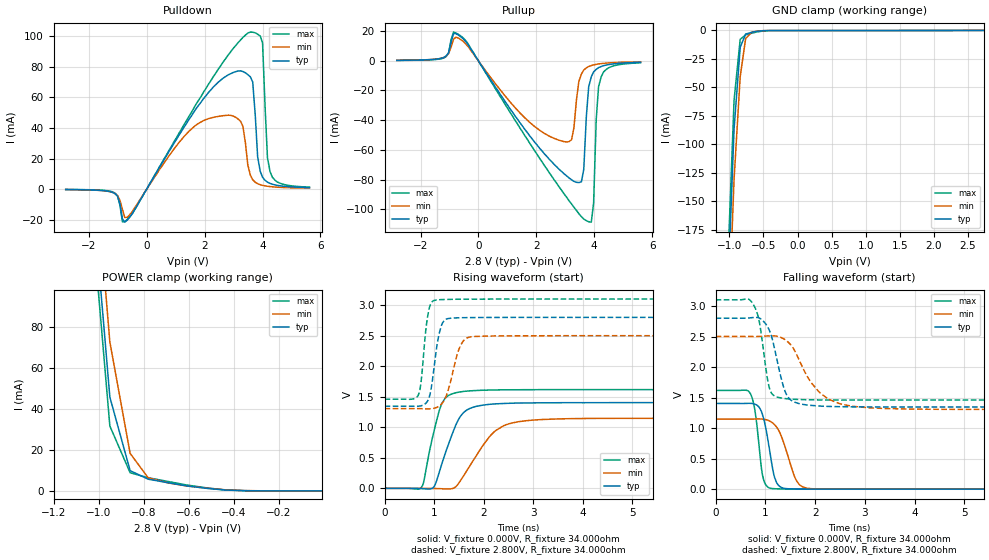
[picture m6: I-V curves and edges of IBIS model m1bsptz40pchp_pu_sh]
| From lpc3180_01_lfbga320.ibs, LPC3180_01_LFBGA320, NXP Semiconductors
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| |   Rev 0.20 IBIS Model Design Automation Generation   |
| |   N O N - S I L I C O N   C O R R E L A T E D   |
| |   This IBIS [Model] is pre-Beta tactical support   |
| |  Note: this IBIS [Model] contains clamp curves generated   |
| |   through simulation which should not be relied upon   |
| mem1bsptz40pchp
|   Bidirectional Pad 2.8
|   3state Output
|   Plain Input
|   1ns Slew Rate control
|   CMOS
| Pull Up Mode (p1=0, p2=0)
[Model]   m1bsptz40pchp_pu_sh | of mem1bsptz40pchp
Model_type   I/O
Polarity   Non-Inverting
Enable   Active-Low
|  Reciever Thresholds
Vinl   = 0.36V
Vinh   = 0.84V
| AC Test Load Conditions
Vref   = 0
Cref   = 1.2e-11
Rref   = 1000000000
Vmeas   = 0.6
| [Process Range]   typical   min   max
| C_comp edge width   400.000ps   400.000ps   400.000ps
| C_comp Tstrobe   40.000fs   40.000fs   40.000fs
C_comp   2.019pF   1.948pF   2.109pF
[Temperature Range]   25   125   -40
[Voltage Range]   2.80V   2.50V   3.10V
[GND Clamp Reference]   0.00V   0.00V   0.00V
[Pulldown Reference]   0.00V   0.00V   0.00V
[POWER Clamp Reference]   2.80V   2.50V   3.10V
[Pullup Reference]   2.80V   2.50V   3.10V
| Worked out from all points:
|   slope of the pulldown table from 0 to 0.42 V, typ, clamps not added: 30.8 ohm
|   slope of the pullup table from 0 to 0.42 V, typ, clamps not added: 32.9 ohm
|   GND clamp passes 1 mA (typ) near -0.61 V on its own axis
|   POWER clamp passes 1 mA (typ) near -0.49 V on its own axis
|   rising waveform, V_fixture 0.000V, R_fixture 34.000ohm: 20-80 % time 380ps typ, 589ps min, 272ps max; typ from 0.001 V to 1.4 V
|   falling waveform, V_fixture 0.000V, R_fixture 34.000ohm: 20-80 % time 183ps typ, 282ps min, 135ps max; typ from 1.4 V to 0.001 V
|   rising waveform, V_fixture 2.800V, R_fixture 34.000ohm: 20-80 % time 155ps typ, 236ps min, 118ps max; typ from 1.35 V to 2.8 V
|   falling waveform, V_fixture 2.800V, R_fixture 34.000ohm: 20-80 % time 260ps typ, 556ps min, 175ps max; typ from 2.8 V to 1.35 V
[GND Clamp]
| ref voltage   0.00V   0.00V   0.00V
|   Voltage   I(typ)   I(min)   I(max)
-2.8V     -3.643A    -3.653A    -3.644A
-1.01V    -211.8mA   -255.9mA   -186.6mA
-930mV    -86.61mA   -130.6mA   -61.25mA
-840mV    -14.85mA   -40.65mA   -7.873mA
-760mV    -3.232mA   -7.1mA     -3.891mA
-670mV    -1.663mA   -1.71mA    -2.461mA
-500mV    -316uA     -247.5uA   -559.8uA
2.73V     -11.67uA   31.94uA    -74.22uA
[Power Clamp]   | Vtable = Vcc - Vpad
| ref voltage   2.80V   2.50V   3.10V
|   Voltage   I(typ)   I(min)   I(max)
-2.82V    3.531A     3.518A     3.546A
-1.03V    149.7mA    178.4mA    134.4mA
-950mV    45.72mA    72.62mA    31.66mA
-860mV    9.875mA    18.31mA    8.866mA
-780mV    5.725mA    6.415mA    6.434mA
-690mV    3.961mA    3.875mA    4.58mA
-610mV    2.472mA    2.439mA    2.908mA
-440mV    442.3uA    569.4uA    500uA
-270mV    46.38uA    47.88uA    58.33uA
-10mV     1.584uA    1.118uA    2.104uA
[Pulldown]
| ref voltage   0.00V   0.00V   0.00V
|   Voltage   I(typ)   I(min)   I(max)
-2.8V     -319.6uA   -345.8uA   -253.3uA
-1.18V    -2.161mA   -2.188mA   -1.788mA
-670mV    -20.27mA   -18.52mA   -19.89mA
2.13V     63.2mA     46.08mA    68.58mA
3.24V     77.42mA    44.42mA    97.59mA
3.58V     73.44mA    9.097mA    102.8mA
3.66V     70.11mA    6.079mA    102.8mA
3.83V     21.16mA    3.502mA    101.4mA
4V        7.734mA    2.421mA    95.8mA
4.17V     4.509mA    1.835mA    20.44mA
4.26V     3.717mA    1.634mA    11.39mA
5.62V     949.5uA    582uA      1.265mA
[Pullup]   | Vtable = Vcc - Vpad
| ref voltage   2.80V   2.50V   3.10V
|   Voltage   I(typ)   I(min)   I(max)
-2.82V    285.4uA    305.9uA    228.1uA
-520mV    14.74mA    12.98mA    15.34mA
2.79V     -73.11mA   -53.54mA   -85.02mA
3.22V     -80.14mA   -53.09mA   -96.45mA
3.47V     -82.02mA   -13.95mA   -103mA
3.64V     -73.04mA   -6.264mA   -106.6mA
3.81V     -17.62mA   -3.881mA   -108.4mA
3.9V      -10.77mA   -3.241mA   -108.7mA
3.98V     -7.53mA    -2.776mA   -95.86mA
4.07V     -5.77mA    -2.424mA   -39.5mA
4.24V     -3.896mA   -1.928mA   -10.84mA
5.6V      -1.048mA   -714.3uA   -1.374mA
[Ramp]
R_load   = 34.000ohm
|   dV/dt(typ)   dV/dt(min)   dV/dt(max)
dV/dt_r   972.011mV/350.000ps   809.309mV/535.000ps   1.110V/250.000ps
dV/dt_f   1.001V/240.000ps   840.428mV/475.000ps   1.123V/165.000ps
[Rising Waveform]  | cubic spline decimation from 2001 points
V_fixture   = 0.000V
R_fixture   = 34.000ohm
|   Time   V(typ)   V(min)   V(max)
0s        719.9uV    560uV      1.036mV
750ps     -3.909mV   873.6uV    25.17mV
995ps     25.56mV    -1.737mV   928.6mV
1.145ns   375.3mV    -5.666mV   1.37V
1.26ns    656.5mV    -9.966mV   1.504V
1.465ns   1.086V     51.77mV    1.571V
1.67ns    1.288V     303.8mV    1.593V
2.14ns    1.378V     868mV      1.61V
2.705ns   1.397V     1.092V     1.615V
10ns      1.404V     1.148V     1.617V
[Falling Waveform]  | cubic spline decimation from 2001 points
V_fixture   = 0.000V
R_fixture   = 34.000ohm
|   Time   V(typ)   V(min)   V(max)
0s        1.404V     1.148V     1.617V
705ps     1.405V     1.148V     1.554V
795ps     1.391V     1.149V     1.261V
940ps     1.226V     1.148V     240.9mV
1.11ns    509mV      1.105V     13.37mV
1.185ns   192.8mV    1.057V     7.983mV
1.28ns    51.33mV    942.1mV    4.991mV
1.615ns   3.648mV    154.8mV    1.748mV
1.84ns    1.805mV    16.04mV    1.336mV
10ns      720.1uV    560.3uV    1.036mV
[Rising Waveform]  | cubic spline decimation from 2001 points
V_fixture   = 2.800V
V_fixture_min = 2.500V
V_fixture_max = 3.100V
R_fixture   = 34.000ohm
|   Time   V(typ)   V(min)   V(max)
0s        1.346V     1.306V     1.46V
675ps     1.345V     1.306V     1.52V
735ps     1.352V     1.305V     1.737V
830ps     1.392V     1.303V     2.578V
890ps     1.469V     1.302V     2.911V
1.045ns   2.275V     1.324V     3.085V
1.21ns    2.754V     1.453V     3.093V
1.525ns   2.794V     2.327V     3.097V
1.74ns    2.797V     2.481V     3.098V
10ns      2.8V       2.5V       3.1V
[Falling Waveform]  | cubic spline decimation from 2001 points
V_fixture   = 2.800V
V_fixture_min = 2.500V
V_fixture_max = 3.100V
R_fixture   = 34.000ohm
|   Time   V(typ)   V(min)   V(max)
0s        2.8V       2.5V       3.1V
735ps     2.809V     2.5V       3.053V
870ps     2.805V     2.502V     2.774V
1.085ns   2.591V     2.51V      1.645V
1.305ns   1.857V     2.488V     1.495V
1.42ns    1.557V     2.433V     1.482V
1.575ns   1.429V     2.288V     1.472V
2.065ns   1.363V     1.605V     1.462V
2.695ns   1.349V     1.366V     1.46V
10ns      1.346V     1.306V     1.46V
